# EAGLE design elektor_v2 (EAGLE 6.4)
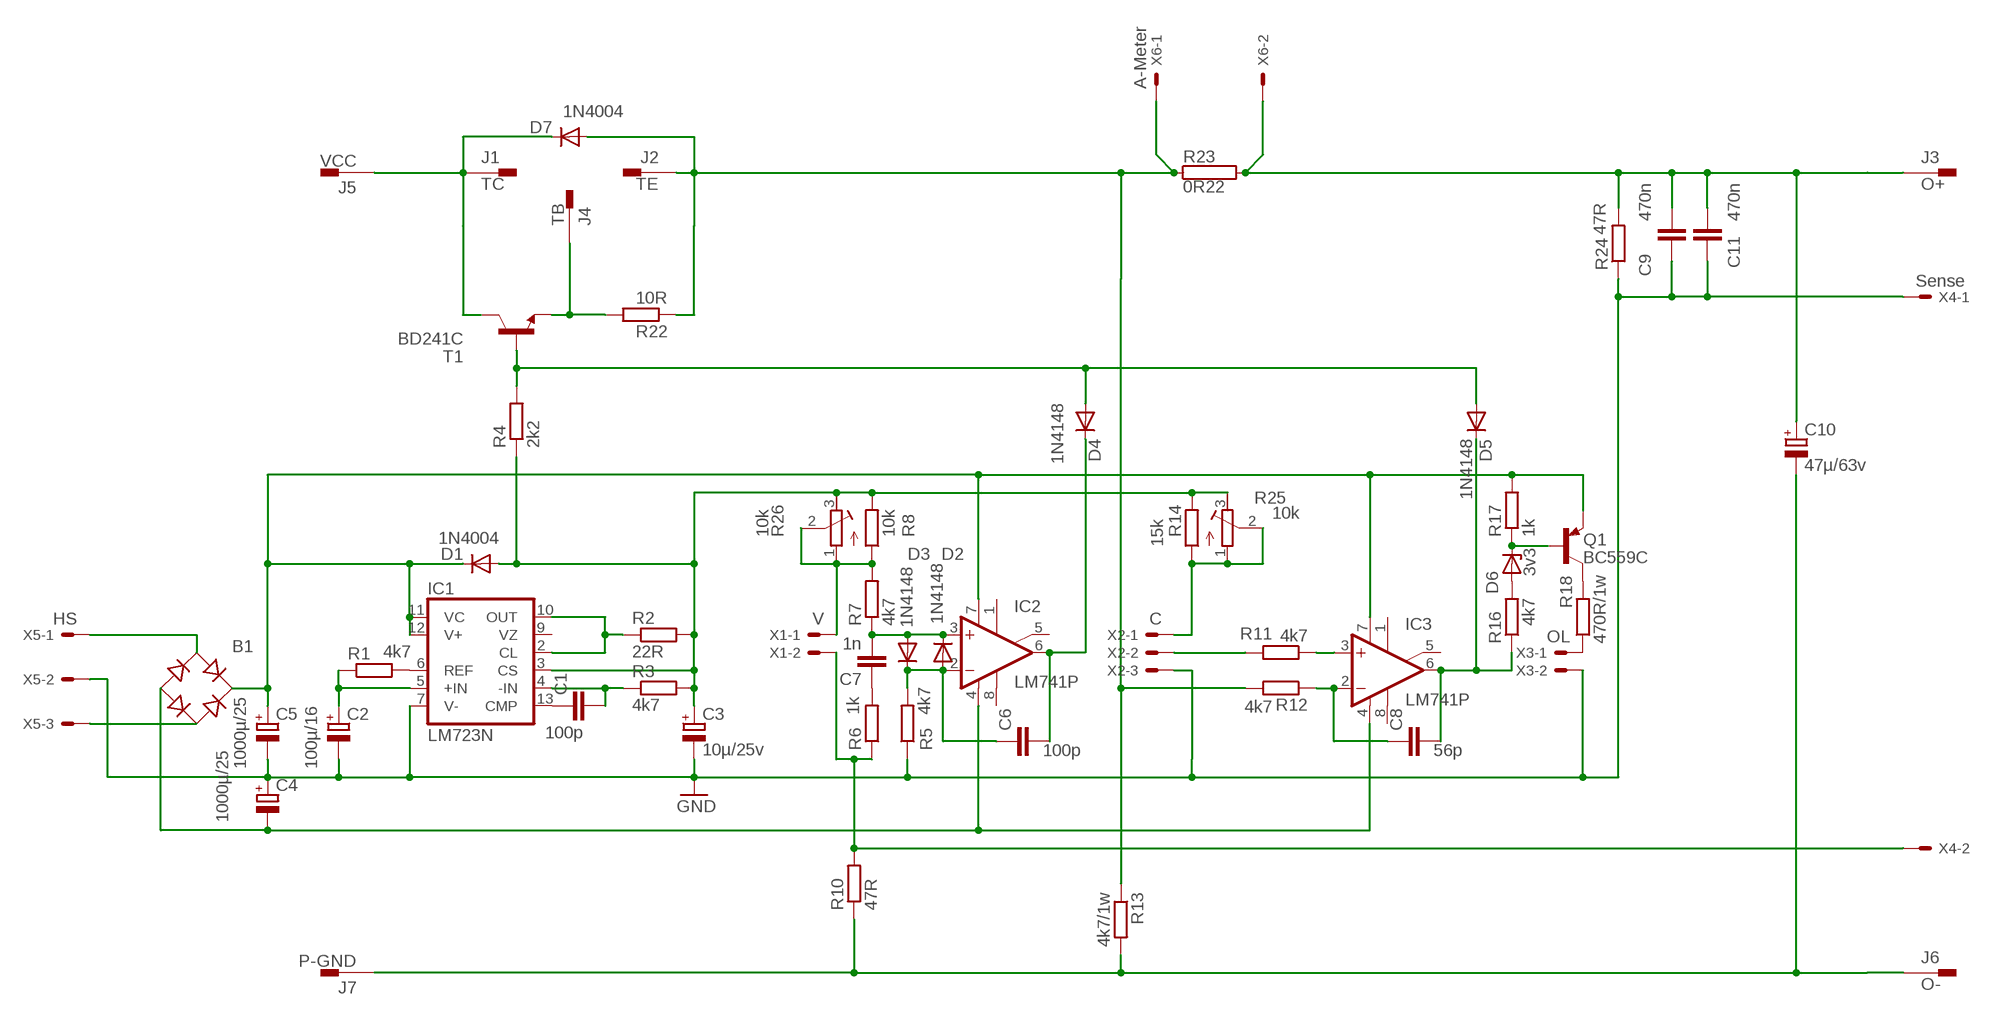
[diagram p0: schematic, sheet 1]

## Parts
B1  RB1A  [RB1A]
C1  100p  C-EU025-024X044  [C025-024X044]
C2  100µ/16  CPOL-EUE2.5-6  [E2,5-6]
C3  10µ/25v  CPOL-EUE2.5-6  [E2,5-6]
C4  1000µ/25  CPOL-EUE5-13  [E5-13]
C5  1000µ/25  CPOL-EUE5-13  [E5-13]
C6  100p  C-EU050-024X044  [C050-024X044]
C7  1n  C-EU050-024X044  [C050-024X044]
C8  56p  C-EU025-024X044  [C025-024X044]
C9  470n  C-EU050-024X044  [C050-024X044]
C10  47µ/63v  CPOL-EUE3.5-8  [E3,5-8]
C11  470n  C-EU050-024X044  [C050-024X044]
D1  1N4004  [DO41-10]
D2  1N4148  1N4148DO35-7  [DO35-7]
D3  1N4148  1N4148DO35-7  [DO35-7]
D4  1N4148  1N4148DO35-7  [DO35-7]
D5  1N4148  1N4148DO35-7  [DO35-7]
D6  3v3  ZENER-DIODEDO34-7  [DO34Z7]
D7  1N4004  [DO41-10]
IC1  LM723N  [DIL14]
IC2  LM741P  [DIL08]
IC3  LM741P  [DIL08]
J1  TC  PIN2F061.040  [F061.040]
J2  TE  PIN2F061.040  [F061.040]
J3  O+  PIN2F061.040  [F061.040]
J4  TB  PIN2F061.040  [F061.040]
J5  VCC  PIN2F061.040  [F061.040]
J6  O-  PIN2F061.040  [F061.040]
J7  P-GND  PIN2F061.040  [F061.040]
Q1  BC559C  [TO92-EBC]
R1  4k7  R-EU_0207/2V  [0207/2V]
R2  22R  R-EU_0207/2V  [0207/2V]
R3  4k7  R-EU_0207/2V  [0207/2V]
R4  2k2  R-EU_0204/7  [0204/7]
R5  4k7  R-EU_0204/7  [0204/7]
R6  1k  R-EU_0204/7  [0204/7]
R7  4k7  R-EU_0207/2V  [0207/2V]
R8  10k  R-EU_0204/7  [0204/7]
R10  47R  R-EU_0204/7  [0204/7]
R11  4k7  R-EU_0204/7  [0204/7]
R12  4k7  R-EU_0204/7  [0204/7]
R13  4k7/1w  R-EU_0204/7  [0204/7]
R14  15k  R-EU_0204/7  [0204/7]
R16  4k7  R-EU_0207/2V  [0207/2V]
R17  1k  R-EU_0207/2V  [0207/2V]
R18  470R/1w  R-EU_0207/2V  [0207/2V]
R22  10R  R-EU_0204/7  [0204/7]
R23  0R22  RKH208-8R  [KH208R-8]
R24  47R  R-EU_0207/2V  [0207/2V]
R25  10k  R-TRIMM64Y  [RTRIM64Y]
R26  10k  R-TRIMM64Y  [RTRIM64Y]
T1  BD241C  TIP31C  [TO220]
X1  V  22-23-2021  [22-23-2021]
X2  C  22-23-2031  [22-23-2031]
X3  OL  22-23-2021  [22-23-2021]
X4  Sense  22-23-2021  [22-23-2021]
X5  HS  22-23-2031  [22-23-2031]
X6  A-Meter  22-23-2021  [22-23-2021]

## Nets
GND: C2.- C3.- C4.+ C5.- C9.1 C11.1 IC1.7(V-) R5.1 R24.1 X2.3 X3.2 X4.1 X5.2
N$1: IC1.6(REF) R1.2
N$2: C2.+ IC1.5(+IN) R1.1
N$3: C1.1 IC1.13(CMP)
N$4: C1.2 IC1.4(-IN) R3.1
N$5: IC1.2(CL) IC1.10(OUT) R2.1
N$6: D7.A J2.A1 J2.A2 R12.2 R13.1 R22.1 R23.1 X6.1
N$7: C6.1 D2.A D3.C IC2.2(-IN) R5.2
N$8: C9.2 C10.+ C11.2 J3.A1 J3.A2 R23.2 R24.2 X6.2
N$9: C7.2 D2.C D3.A IC2.3(+IN) R7.1
N$10: C6.2 D4.C IC2.6(OUT)
N$11: C10.- J6.A1 J6.A2 J7.A1 J7.A2 R10.1 R13.2
N$12: B1.AC1 X5.1
N$13: B1.AC2 X5.3
N$14: B1.+ C5.+ D1.C IC1.11(VC) IC1.12(V+) IC2.7(V+) IC3.7(V+) Q1.E R17.2
N$15: B1.- C4.- IC2.4(V-) IC3.4(V-)
N$16: C7.1 R6.2
N$17: R7.2 R8.1 R26.1(A) R26.2(S) X1.1
N$18: C3.+ D1.A IC1.3(CS) R2.2 R3.2 R4.1 R8.2 R14.2 R25.3(E) R26.3(E)
N$19: R6.1 R10.2 X1.2 X4.2
N$21: C8.2 D5.C IC3.6(OUT) R16.1
N$22: C8.1 IC3.2(-IN) R12.1
N$25: R11.2 X2.2
N$26: R14.1 R25.1(A) R25.2(S) X2.1
N$28: IC3.3(+IN) R11.1
N$29: D6.A R16.2
N$30: D6.C Q1.B R17.1
N$31: Q1.C R18.2
N$32: R18.1 X3.1
N$34: D4.A D5.A R4.2 T1.1(B)
N$35: J4.A1 J4.A2 R22.2 T1.3(E)
N$36: D7.C J1.A1 J1.A2 J5.A1 J5.A2 T1.2(C)
Unconnected: IC1.9(VZ) IC2.1(ON1) IC2.5(ON2) IC2.8(OPT) IC3.1(ON1) IC3.5(ON2) IC3.8(OPT)

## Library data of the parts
B1 = rectifier:RB1A: RECTIFIER 1 A
C1 C6-C9 C11 = rcl:C-EU: CAPACITOR, European symbol
C2-C5 C10 = rcl:CPOL-EU: POLARIZED CAPACITOR, European symbol
D1 D7 = diode:1N4004: DIODE
D2-D5 = diode:1N4148: DIODE
D6 = diode:ZENER-DIODE: Z-Diode
IC1 = linear:*723: Positive VOLTAGE REGULATOR
IC2 IC3 = linear:*741: OP AMP
J1-J7 = con-faston:PIN2: Flachstecker Typ Tyco/Electronics/AMP TAB, FASTON; OC_FARNELL: unknown; OC_NEWARK: unknown
Q1 = transistor-pnp:BC559*: PNP Transistror
R1-R8 R10-R14 R16-R18 R22 R24 = rcl:R-EU_: RESISTOR, European symbol
R23 = resistor-power:R: Power Resitor; OC_FARNELL: unknown; OC_NEWARK: unknown
R25 R26 = rcl:R-TRIMM: Trimm resistor
T1 = transistor:TIP31: NPN Transistor Medium Power Linear Switching Applications Source: http://onsemi.com
X1 X3 X4 X6 = con-molex:22-23-2021: .100" (2.54mm) Center Header - 2 Pin; MF: MOLEX; MPN: 22-23-2021; OC_FARNELL: 1462926; OC_NEWARK: 25C3832
X2 X5 = con-molex:22-23-2031: .100" (2.54mm) Center Header - 3 Pin; MF: MOLEX; MPN: 22-23-2031; OC_FARNELL: 1462950; OC_NEWARK: 30C0862

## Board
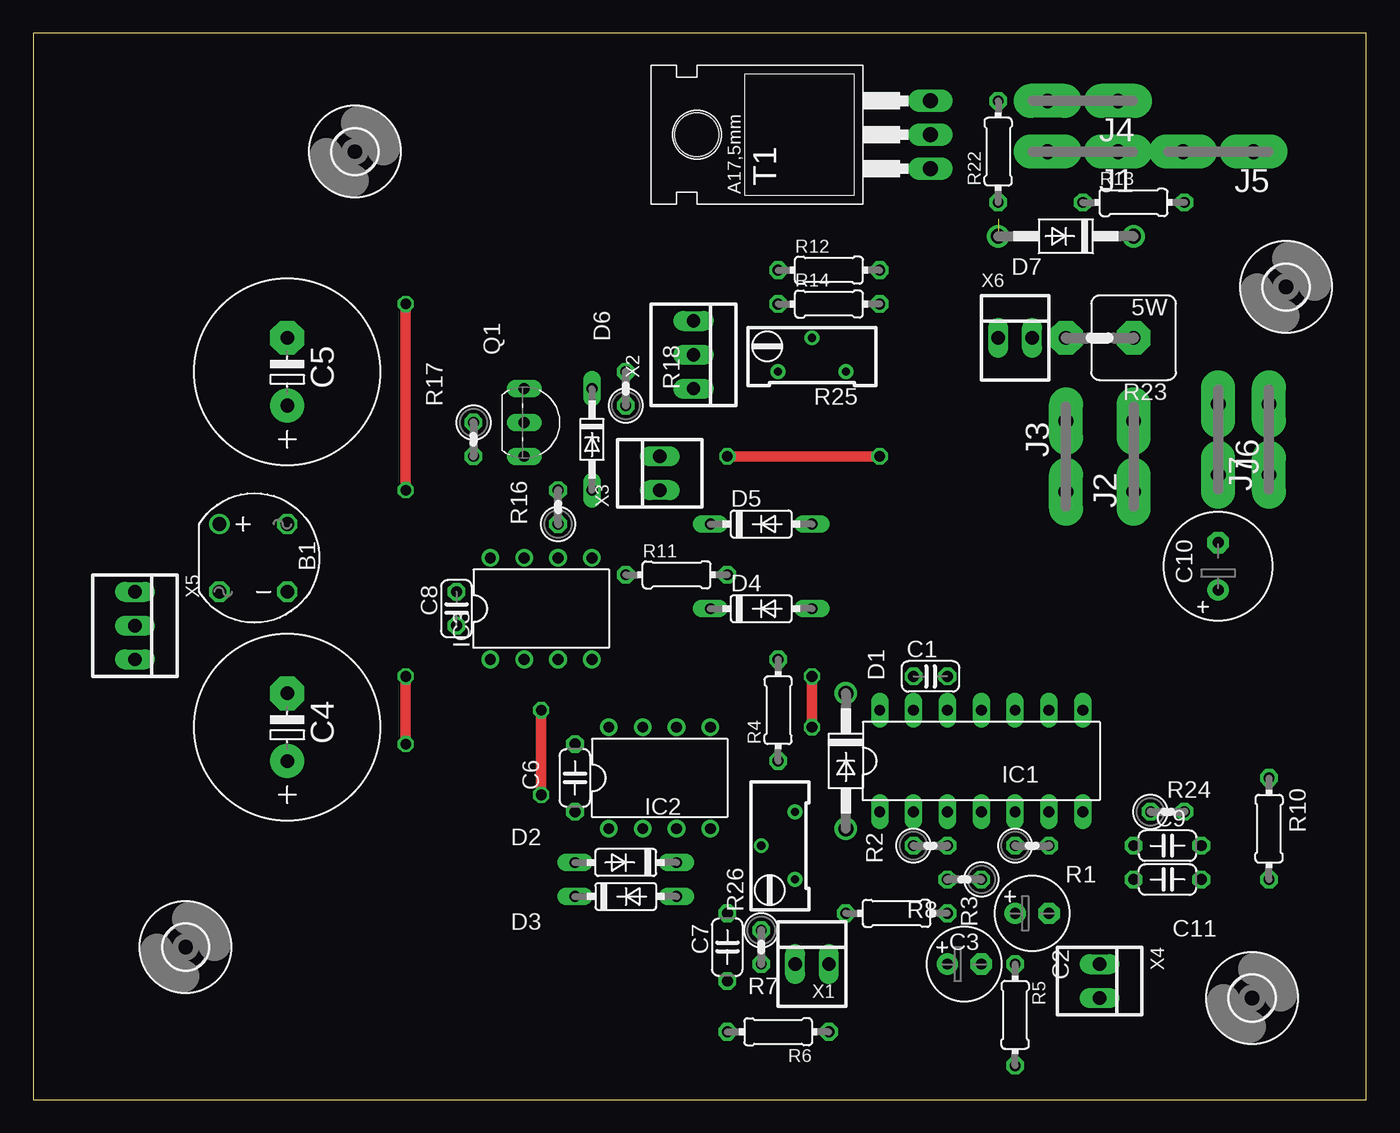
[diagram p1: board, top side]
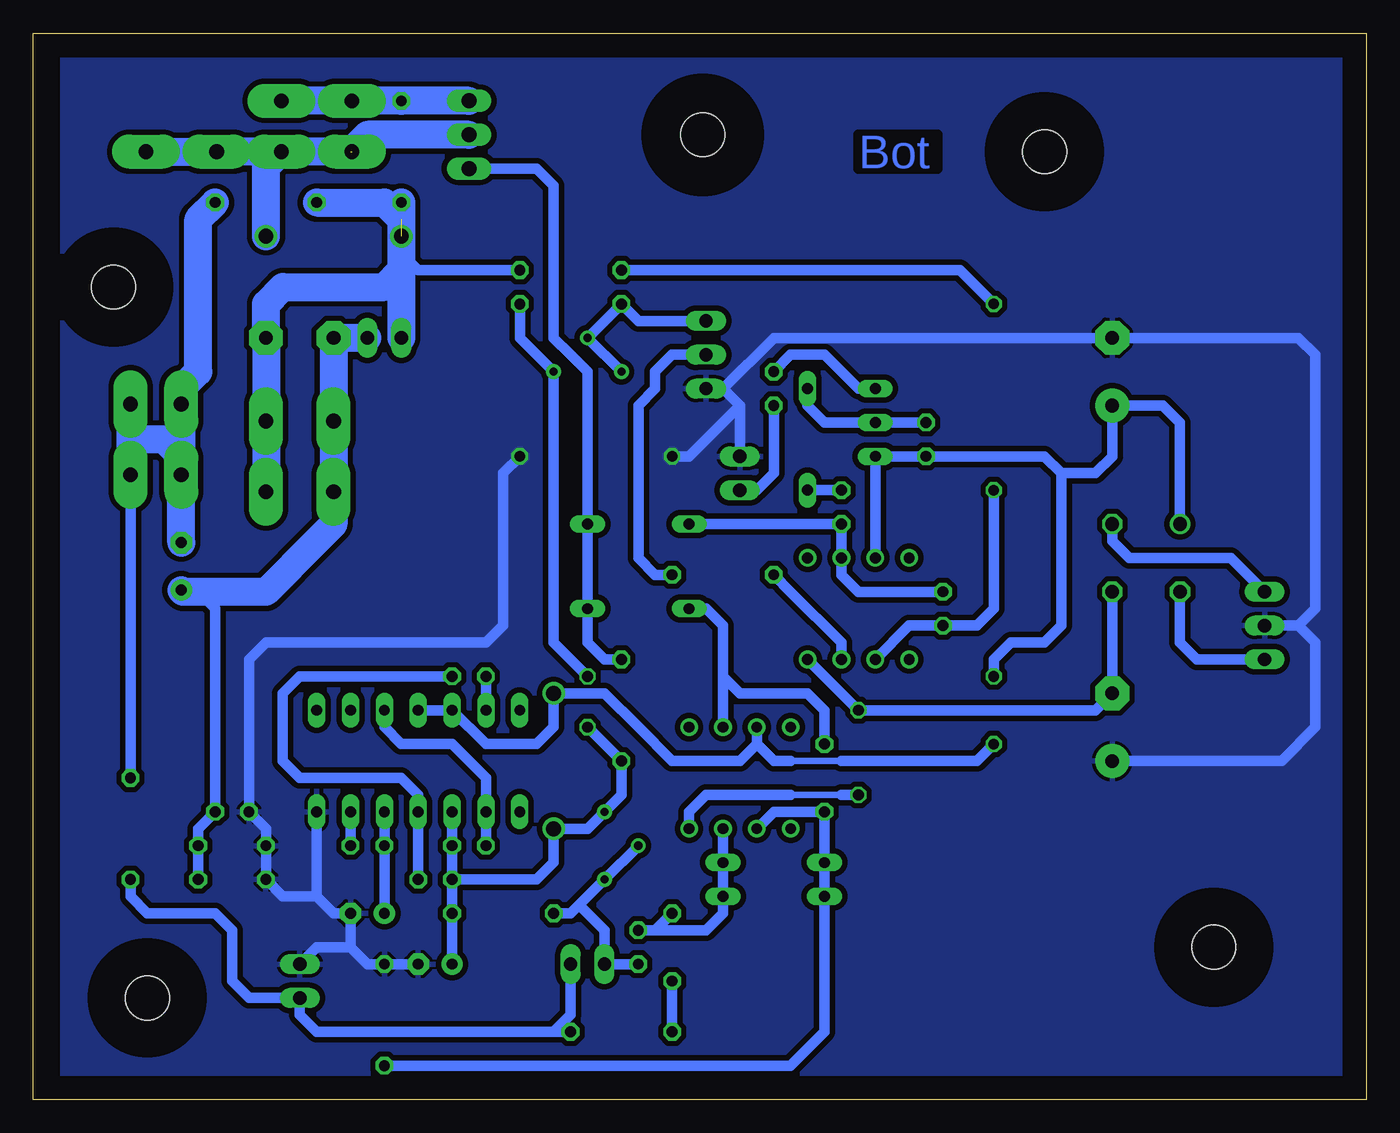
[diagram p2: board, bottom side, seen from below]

Size 100 x 80 mm. Coordinates in mm from the lower left corner, seen from the top.
Outline: 0,0 100,0 100,80 0,80 0,0
Copper layers (1*16): Top 0.035mm / dielectric 2.5mm / Bottom 0.035mm
Design rules "default *": minimum track width 12mil, minimum drill 24mil, track to track 10mil, track to pad 8mil, pad to pad 8mil, via to via 8mil, smd to smd 8mil, copper to edge 70mil, drill to drill 8mil, minimum pad ring 10mil, minimum via ring 8mil, stop-mask expansion 4mil, vias tented up to drill 0mil, thermal gap 10mil

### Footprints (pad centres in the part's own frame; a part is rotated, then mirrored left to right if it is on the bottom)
RB1A = drill 1.016: + -2.54,2.54 | drill 1.016 octagon: - 2.54,-2.54; AC1 2.54,2.54; AC2 -2.54,-2.54
C025-024X044 = drill 0.813 octagon: 1 -1.27,0; 2 1.27,0
E2,5-6 = drill 0.813 pad 1.6: + -1.27,0 | drill 0.813 pad 1.6 octagon: - 1.27,0
E5-13 = drill 1.016 pad 2.54: + -2.54,0 | drill 1.016 pad 2.54 octagon: - 2.54,0
C050-024X044 = drill 0.813 octagon: 1 -2.54,0; 2 2.54,0
E3,5-8 = drill 0.813 pad 1.6: + -1.778,0 | drill 0.813 pad 1.6 octagon: - 1.778,0
DO41-10 = drill 1.118: A 5.08,0; C -5.08,0
DO35-7 = drill 0.813 long: A 3.81,0; C -3.81,0
DO34Z7 = drill 0.813 long: A 3.81,0; C -3.81,0
DIL14 = drill 0.813 long: 1 -7.62,-3.81; 2 -5.08,-3.81; 3 -2.54,-3.81; 4 0,-3.81; 5 2.54,-3.81; 6 5.08,-3.81; 7 7.62,-3.81; 8 7.62,3.81; 9 5.08,3.81; 10 2.54,3.81; 11 0,3.81; 12 -2.54,3.81; 13 -5.08,3.81; 14 -7.62,3.81
DIL08 = drill 0.813 pad 1.27: 1 -3.81,-3.81; 2 -1.27,-3.81; 3 1.27,-3.81; 4 3.81,-3.81; 5 3.81,3.81; 6 1.27,3.81; 7 -1.27,3.81; 8 -3.81,3.81
F061.040 = drill 1.1 pad 2.54 long: A1 -2.65,0; A2 2.65,0
TO92-EBC = drill 0.813 long: B 0,-1.27; C -2.54,-1.27; E 2.54,-1.27
0207/2V = drill 0.813 octagon: 1 -1.27,0; 2 1.27,0
0204/7 = drill 0.813 octagon: 1 -3.81,0; 2 3.81,0
KH208R-8 = drill 1.016 pad 2.54 octagon: 1 -2.54,0; 2 2.54,0
RTRIM64Y = drill 0.61: 1 0,-2.54; 2 -2.54,0; 3 0,2.54
TO220 = drill 1.118 long: 1 -2.54,-6.35; 2 0,-6.35; 3 2.54,-6.35 | hole 3.302: 0,11.176
3,3 = hole 3.3: 0,0
22-23-2021 = drill 1 long: 1 -1.27,0; 2 1.27,0
22-23-2031 = drill 1 long: 1 -2.54,0; 2 0,0; 3 2.54,0

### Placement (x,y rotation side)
B1  16.51,40.64 0 top
C1  67.31,31.75 0 top
C2  74.93,13.97 0 top
C3  69.85,10.16 0 top
C4  19.05,27.94 90 top
C5  19.05,54.61 90 top
C6  40.64,24.13 90 top
C7  52.07,11.43 90 top
C8  31.75,36.83 90 top
C9  85.09,19.05 0 top
C10  88.9,40.01 90 top
C11  85.09,16.51 0 top
D1  60.96,25.4 270 top
D2  44.45,17.78 180 top
D3  44.45,15.24 0 top
D4  54.61,36.83 0 top
D5  54.61,43.18 0 top
D6  41.91,49.53 270 top
D7  77.47,64.77 180 top
IC1  71.12,25.4 0 top
IC2  46.99,24.13 0 top
IC3  38.1,36.83 0 top
J1  78.74,71.12 180 top
J2  82.55,48.26 90 top
J3  77.47,48.26 90 top
J4  78.74,74.93 180 top
J5  88.9,71.12 180 top
J6  88.9,49.53 90 top
J7  92.71,49.53 90 top
Q1  38.1,50.8 270 top
R1  74.93,19.05 0 top
R2  67.31,19.05 0 top
R3  69.85,16.51 180 top
R4  55.88,29.21 90 top
R5  73.66,6.35 270 top
R6  55.88,5.08 180 top
R7  54.61,11.43 270 top
R8  64.77,13.97 0 top
R10  92.71,20.32 270 top
R11  48.26,39.37 0 top
R12  59.69,62.23 0 top
R13  82.55,67.31 0 top
R14  59.69,59.69 0 top
R16  39.37,44.45 90 top
R17  33.02,49.53 270 top
R18  44.45,53.34 90 top
R22  72.39,71.12 90 top
R23  80.01,57.15 180 top
R24  85.09,21.59 0 top
R25  58.42,54.61 270 top
R26  57.15,19.05 0 top
T1  60.96,72.39 90 top
U$1  [3,3]  11.43,11.43 0 top
U$2  [3,3]  91.44,7.62 0 top
U$3  [3,3]  24.13,71.12 0 top
U$4  [3,3]  93.98,60.96 0 top
X1  58.42,10.16 0 top
X2  49.53,55.88 270 top
X3  46.99,46.99 90 top
X4  80.01,8.89 270 top
X5  7.62,35.56 270 top
X6  73.66,57.15 0 top

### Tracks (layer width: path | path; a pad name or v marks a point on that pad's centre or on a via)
GND  (via drill 0.8)
  Top 0.8: v52.07,48.26 v63.5,48.26
  Bottom 0.8: IC1.7 78.74,15.24 | 78.74,15.24 77.47,13.97 C2.- 76.2,11.43 | C3.- R5.1 | R5.1 74.93,10.16 | 74.93,10.16 76.2,11.43 | C4.+ 6.35,25.4 3.81,27.94 3.81,34.29 5.08,35.56 | 5.08,35.56 X5.2 | 5.08,35.56 3.81,36.83 3.81,55.88 5.08,57.15 C5.- 30.48,57.15 44.45,57.15 48.26,53.34 | X3.2 46.99,50.8 | 46.99,50.8 46.99,52.07 | 46.99,52.07 48.26,53.34 | 48.26,53.34 X2.3 | 78.74,15.24 81.28,15.24 C11.1 C9.1 82.55,20.32 R24.1 83.82,33.02 82.55,34.29 73.66,34.29 66.04,34.29 64.77,35.56 64.77,46.99 v63.5,48.26 | X4.1 78.74,11.43 76.2,11.43 | X3.2 46.99,50.8 | 46.99,50.8 46.99,52.07 | 46.99,52.07 50.8,48.26 v52.07,48.26 | X3.2 46.99,52.07 | 46.99,52.07 48.26,53.34 | R5.1 74.93,10.16
  pour Bottom (isolate 0.4): 1.27,1.27 1.27,78.74 97.79,78.74 97.79,1.27
N$1
  Bottom 0.8: IC1.6 R1.2
N$2
  Bottom 0.8: C2.+ R1.1 IC1.5
N$3
  Bottom 0.8: IC1.13 C1.1
N$4
  Bottom 0.8: R3.1 IC1.4 71.12,22.86 72.39,24.13 80.01,24.13 81.28,25.4 81.28,30.48 80.01,31.75 73.66,31.75 C1.2
N$5
  Bottom 0.8: R2.1 IC1.2 66.04,24.13 68.58,26.67 72.39,26.67 73.66,27.94 IC1.10
N$6  (1 unrouted)
  Bottom 0.8: R12.2 71.12,62.23 72.39,63.5
  Bottom 2.1: R22.1 72.39,66.04 | 72.39,66.04 72.39,63.5 72.39,62.23 | R13.1 73.66,67.31 72.39,66.04 | 72.39,62.23 X6.1 | 72.39,62.23 73.66,60.96 81.28,60.96 82.55,59.69 R23.1 J2.A2 J2.A1
N$7
  Bottom 0.8: IC2.2 44.45,21.59 C6.1 D2.A D3.C 40.64,10.16 40.64,5.08 43.18,2.54 R5.2
N$8
  Bottom 0.8: C11.2 C9.2 87.63,20.32 R24.2 86.36,36.83 87.63,38.1
  Bottom 2.1: X6.2 R23.2 J3.A2 J3.A1 77.47,43.18 78.74,41.91 82.55,38.1 87.63,38.1 88.77,38.1 C10.+
N$9
  Bottom 0.8: IC2.3 D2.C D3.A 48.26,13.97 49.53,12.7 53.34,12.7 | R7.1 53.34,12.7 | 53.34,12.7 C7.2
N$10
  Bottom 0.8: IC2.6 48.26,29.21 48.26,31.75 | 48.26,31.75 48.26,35.56 49.53,36.83 D4.C | C6.2 40.64,29.21 41.91,30.48 46.99,30.48 48.26,31.75
N$11
  Bottom 0.8: R10.1 J7.A1
  Bottom 2.1: J6.A1 C10.- 88.9,48.26 90.17,49.53 92.71,49.53 | J6.A1 J6.A2 | J6.A2 J6.A1 | J7.A1 92.71,49.53 | 92.71,49.53 J7.A2 | J6.A2 88.9,53.34 87.63,54.61 87.63,66.04 R13.2
N$12
  Bottom 0.8: B1.AC1 19.05,41.91 17.78,40.64 10.16,40.64 X5.1
N$13
  Bottom 0.8: X5.3 12.7,33.02 13.97,34.29 B1.AC2
N$14  (via drill 0.8)
  Top 0.8: v27.94,26.67 v27.94,31.75
  Bottom 0.5: 43.18,25.4 39.37,25.4
  Bottom 0.8: B1.+ 13.97,50.8 15.24,52.07 C5.+ 19.05,48.26 20.32,46.99 22.86,46.99 | IC1.11 IC1.12 66.04,26.67 62.23,26.67 60.96,27.94 D1.C 57.15,30.48 54.61,27.94 52.07,25.4 46.99,25.4 45.72,26.67 | 45.72,26.67 IC2.7 45.72,26.67 | 45.72,26.67 44.45,25.4 43.18,25.4 | IC3.7 Q1.E R17.2 30.48,48.26 24.13,48.26 22.86,46.99 | 39.37,25.4 29.21,25.4 v27.94,26.67 | v27.94,31.75 27.94,33.02 26.67,34.29 24.13,34.29 22.86,35.56 22.86,46.99
N$15  (via drill 0.8)
  Top 0.8: v38.1,29.21 v38.1,22.86
  Bottom 0.5: 39.37,22.86 43.18,22.86
  Bottom 0.8: B1.- C4.- 20.32,29.21 v38.1,29.21 40.64,31.75 IC3.4 | 43.18,22.86 49.53,22.86 50.8,21.59 IC2.4 | 39.37,22.86 v38.1,22.86
N$16
  Bottom 0.8: R6.2 C7.1
N$17
  Bottom 0.8: R26.2 R26.1 59.05,14.61 | R8.1 59.69,13.97 59.05,14.61 | R7.2 X1.1 57.15,12.7 59.05,14.61
N$18  (via drill 0.8)
  Top 0.8: v58.42,31.75 v58.42,27.94
  Bottom 0.8: C3.+ R8.2 | R8.2 R3.2 | R3.2 R2.2 IC1.3 | R3.2 62.23,16.51 60.96,17.78 D1.A 59.69,20.32 58.42,20.32 R26.3 | 55.88,22.86 R4.1 v58.42,27.94 | 55.88,22.86 R26.3 | v58.42,31.75 60.96,34.29 60.96,40.64 60.96,52.07 R25.3 62.23,55.88 63.5,57.15 R14.2 | R8.2 R3.2 | R26.3 55.88,22.86
N$19
  Bottom 0.8: R6.1 60.96,5.08 | 60.96,5.08 76.2,5.08 78.74,5.08 80.01,6.35 X4.2 83.82,7.62 85.09,8.89 85.09,12.7 86.36,13.97 91.44,13.97 92.71,15.24 R10.2 | X1.2 59.69,6.35 60.96,5.08
N$21
  Bottom 0.8: D5.C R16.1 IC3.6 39.37,39.37 38.1,38.1 C8.2
N$22  (via drill 0.8)
  Top 0.8: v27.94,59.69 v27.94,45.72
  Bottom 0.8: IC3.2 34.29,35.56 C8.1 30.48,35.56 29.21,35.56 27.94,36.83 27.94,44.45 | R12.1 30.48,62.23 v27.94,59.69 | 27.94,44.45 v27.94,45.72 27.94,44.45
N$25
  Bottom 0.8: R11.2 53.34,39.37 54.61,40.64 54.61,52.07 53.34,53.34 53.34,54.61 52.07,55.88 X2.2
N$26
  Bottom 0.8: X2.1 54.61,58.42 R14.1 R25.2 R25.1
N$28
  Bottom 0.8: IC3.3 39.37,34.29 43.18,38.1 R11.1
N$29
  Bottom 0.8: R16.2 D6.A
N$30
  Bottom 0.8: D6.C 41.91,52.07 40.64,50.8 Q1.B R17.1
N$31
  Bottom 0.8: Q1.C 38.1,53.34 40.64,55.88 43.18,55.88 R18.2
N$32
  Bottom 0.8: X3.1 45.72,45.72 44.45,46.99 R18.1
N$34
  Bottom 0.8: D4.A D5.A 58.42,54.61 59.69,55.88 60.96,57.15 60.96,62.23 60.96,68.58 62.23,69.85 T1.1 | D4.A 58.42,34.29 | 58.42,34.29 D4.A | 58.42,34.29 57.15,33.02 R4.2
N$35
  Bottom 2.1: T1.3 R22.2 75.82,74.93 J4.A2 J4.A1
N$36  (1 unrouted)
  Bottom 2.1: T1.2 74.93,72.39 76.2,71.12 J1.A1 | D7.C 82.55,69.96 J1.A1 | J5.A1 J5.A2 J1.A1

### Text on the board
Bottom: Bot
